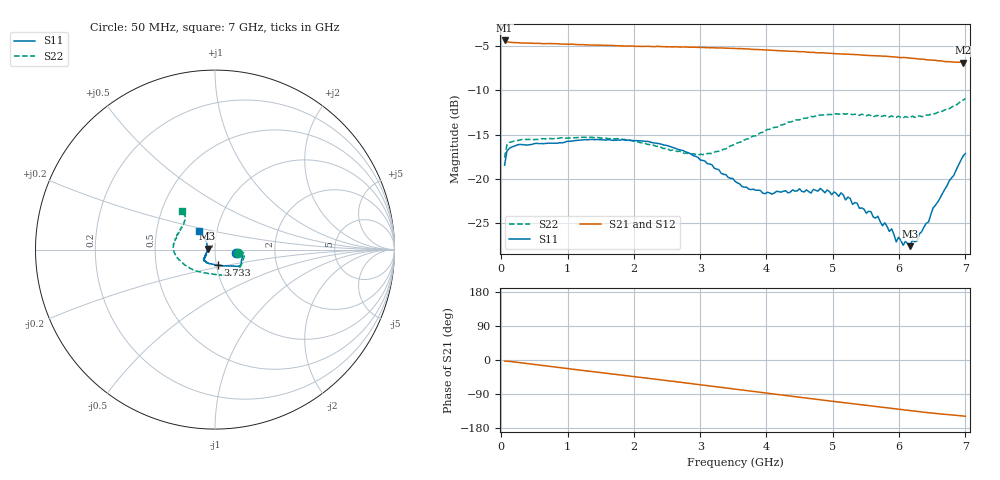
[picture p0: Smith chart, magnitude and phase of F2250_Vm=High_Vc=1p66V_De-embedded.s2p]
! Integrated Device Technology
! Corporate Headquarters
! 6024 Silver Creek Valley Road
! San Jose, CA 95138  USA
! Phone:  1-408-284-8200
! Toll Free:  1-800-223-1366
! Webpage:  http://www.idt.com/
! Timing and RF Division
! 515 Groton Road, Suite 102
! Westford, MA 01886-6024
! Device:  F2250
! Description: Voltage Variable RF Attenuator
! Frequency:  50.0 -  6000.00 MHz
! Package:  3x3 mm Thin QFN Plastic Package: 16 pin
! Ports:  2 RF, 3 DC
!  Pin  1  = GND
!  Pin  2  = NC
!  Pin  3  = RF1  = Port 1
!  Pin  4  = NC
!  Pin  5  = GND
!  Pin  6  = GND
!  Pin  7  = GND
!  Pin  8  = GND
!  Pin  9  = NC
!  Pin 10  = RF2  = Port 2
!  Pin 11  = NC
!  Pin 12  = GND
!  Pin 13  = GND
!  Pin 14  = VCNTRL
!  Pin 15  = VDD
!  Pin 16  = VMODE
! Vcntrl:  1.660 Volts
! Vmode:  +3.300 Volts
! Vdd:  +3.30  Volts
! Current:  1.328 mA
! Data:  The device was measured on a the F2250 evaluation board which has
!  individual transmission lines to the RF pins.  Data was collected
!  using a calibrated network analyzer.  The evaluation board was
!  de-embedded using a TRL calibration technique.
!  The reference plane is the edge of the package pin.
! Misc:  SN 10
!  Action Tracker AT0258
! Date Measured:  2014-11-26
! Date:  2015-10-15  MJV
! Note:
!  Integrated Device Technology supplies this data as a sample of measured
!  data at the package pin for this product.  Your particular data for this
!  product may vary.
!  Data was taken at 25 degrees C.
!  Integrated Device Technology reserves the right to change this data at anytime.
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# GHz S dB R 50
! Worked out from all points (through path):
!   201 points, 50 MHz to 7 GHz, reference 50 ohm
!   highest |S21| = -4.34 dB at 50 MHz (marker M1); lowest = -6.8 dB at 6.965 GHz (marker M2)
!   group delay of S21, straight-line fit = 59.5 ps
!   lowest |S11| = -27.7 dB at 6.166 GHz (marker M3), VSWR 1.09, Z = 46.1 + j0.539 ohm
!   |S11| at or under -10 dB: start of sweep to end of sweep
!   |S22| runs from -17.6 to -10.9 dB; largest |S21 - S12| = 0.0025
!   S11 on the Smith chart (normalised r, x): 50 MHz: 1.27, -0.04; 3.733 GHz: 1.01, -0.18; 7 GHz: 0.82, +0.18
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0.05  -18.47 -8.3  -4.34 -2.9  -4.35 -2.9  -17.63 -8.5
0.08475  -16.89 -5.3  -4.49 -3.1  -4.49 -3.1  -16.17 -6.1
0.2585  -16.14 -7.9  -4.60 -6.5  -4.60 -6.5  -15.66 -11.4
1.2315  -15.59 -28.4  -4.81 -27.6  -4.82 -27.6  -15.30 -43.8
2.37825  -16.03 -36.3  -5.02 -51.7  -5.04 -51.7  -16.33 -71.1
2.969  -17.62 -43.7  -5.12 -64.5  -5.10 -64.6  -17.31 -97.2
3.525  -20.30 -66.7  -5.26 -76.9  -5.25 -76.9  -16.11 -130.0
3.7335  -21.19 -80.4  -5.30 -81.6  -5.32 -81.6  -15.47 -140.3
4.081  -21.76 -103.6  -5.45 -89.2  -5.44 -89.2  -14.33 -155.7
4.7065  -21.22 -131.8  -5.68 -102.8  -5.69 -102.8  -12.98 -174.4
5.1235  -21.61 -140.8  -5.86 -111.7  -5.88 -111.7  -12.66 175.3
5.6795  -24.27 -150.4  -6.07 -123.4  -6.07 -123.5  -12.84 162.0
5.85325  -25.98 -158.4  -6.17 -127.0  -6.19 -127.1  -13.00 156.6
5.888  -25.69 -159.6  -6.19 -127.8  -6.21 -127.8  -12.89 156.7
5.9575  -27.17 -165.8  -6.22 -129.1  -6.24 -129.2  -13.06 153.8
5.99225  -26.65 -170.3  -6.25 -130.0  -6.25 -130.1  -12.91 153.4
6.06175  -27.56 -175.3  -6.26 -131.3  -6.27 -131.4  -13.12 150.6
6.166  -27.65 171.9  -6.34 -133.5  -6.35 -133.6  -13.06 147.3
6.444  -24.91 141.8  -6.54 -139.0  -6.55 -139.2  -12.80 138.7
6.5135  -23.31 136.7  -6.58 -140.3  -6.58 -140.5  -12.65 136.3
6.96525  -17.45 130.3  -6.84 -147.9  -6.82 -148.0  -11.10 130.6
7  -17.15 130.2  -6.83 -148.4  -6.84 -148.5  -10.94 129.9
